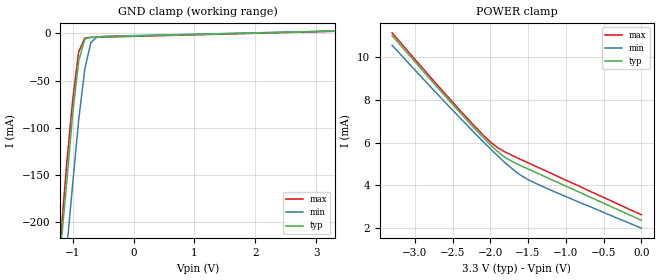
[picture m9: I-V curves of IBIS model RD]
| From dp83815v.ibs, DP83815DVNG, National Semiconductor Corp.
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|   Model RD
[Model]   RD
Model_type   Input
Polarity   Non-Inverting
Enable   Active-High
Vinl =   0.80V
Vinh =   2.00V
Vmeas =   1.50V
Cref =  20.00pF
Rref = 100.00k
C_comp   5.00pF   5.00pF   5.00pF
[Temperature Range]   25.00   0.14k   0.000
[Voltage Range]   3.30V   3.00V   3.60V
[GND_clamp]
| voltage   I(typ)   I(min)   I(max)
-3.3V     -1.96A     -2.02A     -1.95A
-1.2V     -230mA     -300mA     -220mA
-1.1V     -160mA     -230mA     -140mA
-1V       -85.43mA   -160mA     -71.07mA
-900mV    -29.09mA   -91.01mA   -19.38mA
-800mV    -6.06mA    -37.6mA    -5.1mA
-700mV    -4.08mA    -9.61mA    -4.36mA
-600mV    -3.86mA    -3.9mA     -4.19mA
3.3V      2.37mA     2.44mA     2.14mA
[POWER_clamp]
| voltage   I(typ)   I(min)   I(max)
-3.3V     11.01mA    10.56mA    11.14mA
-2.6V     8.19mA     7.9mA      8.3mA
-2.2V     6.64mA     6.43mA     6.75mA
-2V       5.91mA     5.72mA     6.04mA
-1.9V     5.58mA     5.38mA     5.76mA
-1.8V     5.3mA      5.05mA     5.56mA
-1.6V     4.93mA     4.48mA     5.22mA
-1.4V     4.61mA     4.1mA      4.9mA
0V        2.37mA     2mA        2.63mA
